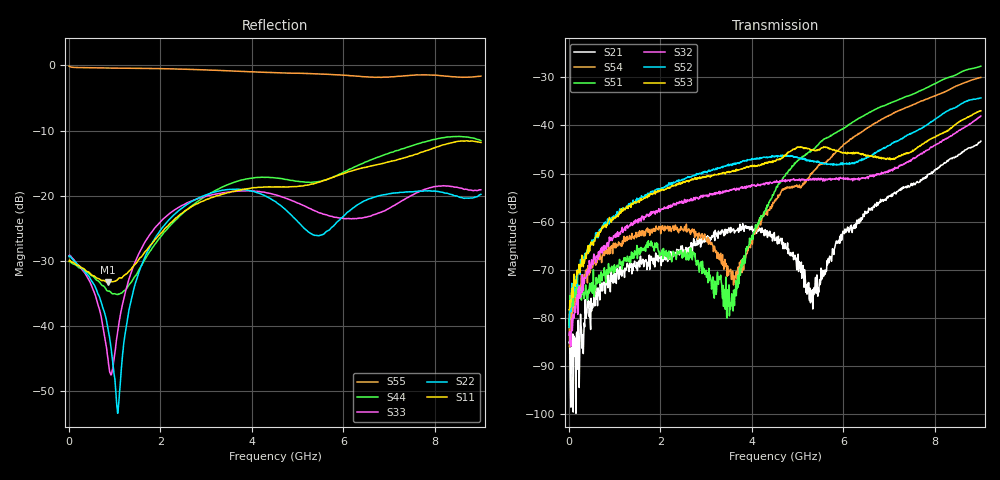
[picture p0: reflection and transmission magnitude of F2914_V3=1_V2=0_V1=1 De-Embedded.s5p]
! Integrated Device Technology
! Corporate Headquarters
! 6024 Silver Creek Valley Road
! San Jose, CA 95138  USA
! Phone:  1-408-284-8200
! Toll Free:  1-800-223-1366
! Webpage:  http://www.idt.com/
! Timing and RF Division
! 515 Groton Road, Suite 102
! Westford, MA 01886-6024
! Device:  F2914
! Description: High Reliability SP4T RF Switch
! Frequency:  0.05 -  8.GHz
! Package:  4x4 mm Thin QFN Plastic Package: 24 pin
! Ports:  5 RF,  5 DC
!  Pin  1  = GND
!  Pin  2  = GND
!  Pin  3  = GND
!  Pin  4  = GND
!  Pin  5  = RF4  =  Port 4
!  Pin  6  = GND
!  Pin  7  = GND
!  Pin  8  = RF3  =  Port 3
!  Pin  9  = GND
!  Pin 10  = GND
!  Pin 11  = RF2  =  Port 2
!  Pin 12  = GND
!  Pin 13  = GND
!  Pin 14  = RF1  =  Port 1
!  Pin 15  = GND
!  Pin 16  = Vcc
!  Pin 17  = V1
!  Pin 18  = V2
!  Pin 19  = V3
!  Pin 20  = VSSext
!  Pin 21  = GND
!  Pin 22  = RFC  =  Port 5
!  Pin 23  = GND
!  Pin 24  = GND
! Voltage:  VDD  =  +3.30 Volts
!  VSSEXT =  0.00 Volts
! Current:  IDD  = 330  uA
! State:  All OFF
! V1:  Logic HIGH
! V2:  Logic LOW
! V3:  Logic HIGH
! Data:  The device was measured on the F291x evaluation board which has
!  individual transmission lines to the RF pins.  Data was collected
!  using a calibrated network analyzer.  The input lines were
!  modeled using Automatic Fixture Removal (AFR) from Keysight.
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# Hz S  dB  R 50
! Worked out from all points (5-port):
!   900 points, 10 MHz to 9 GHz, reference 50 ohm
!   strongest paths, dB at 10 MHz, 2.26 GHz, 4.51 GHz, 6.76 GHz, 9 GHz:
!     S53: -78.3, -52.6, -47.3, -46.6, -37.0
!     S52: -81.9, -52.3, -46.5, -45.2, -34.3
!     S32: -83.6, -56.8, -51.7, -50.1, -38.0
!     S51: -82.0, -67.6, -53.6, -36.4, -27.7
!     S54: -79.3, -61.4, -55.6, -39.1, -30.0
!     S21: -85.1, -67.6, -63.8, -56.2, -43.3
!   lowest |S11| = -33.3 dB at 850 MHz (marker M1), VSWR 1.04, Z = 48.6 + j1.6 ohm
!   |S11| at or under -10 dB: start of sweep to end of sweep
